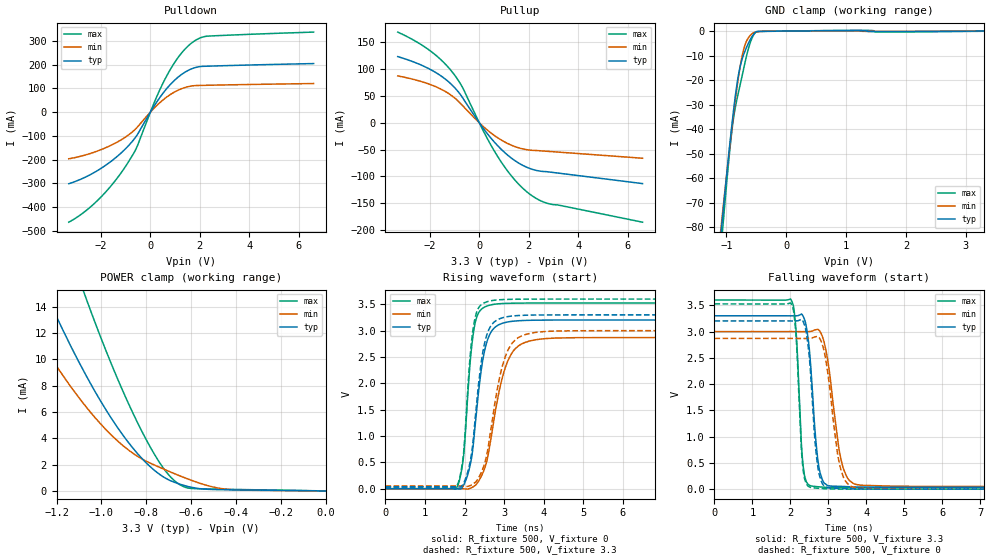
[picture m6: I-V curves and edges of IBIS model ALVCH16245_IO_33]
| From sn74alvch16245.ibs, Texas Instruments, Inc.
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[Model]   ALVCH16245_IO_33
Model_type  I/O
Vinl=0.8
Vinh=2.0
Enable   Active-Low
Vref =   0
Rref =   500
Cref =   50p
Vmeas =   1.5
| variable   typ   min   max
C_comp   8.05pF   6.87pF   9.23pF
| C_pullup   9.24pF   7.49pF   10.37pF
| C_pulldown   11.78pF   9.38pF   15.22pF
| C_tri-state   8.05pF   6.87pF   9.23pF
[Temperature Range]   40   100   -40
| Ambient temperature   25   85   -40
[Voltage range]   3.3   3   3.6
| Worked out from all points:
|   slope of the pulldown table from 0 to 0.495 V, typ, clamps not added: 6.36 ohm
|   slope of the pullup table from 0 to 0.495 V, typ, clamps not added: 16.5 ohm
|   GND clamp passes 1 mA (typ) near -0.54 V on its own axis
|   POWER clamp passes 1 mA (typ) near -0.72 V on its own axis
|   rising waveform, R_fixture 500, V_fixture 0: 20-80 % time 302ps typ, 451ps min, 214ps max; typ from 0 V to 3.2 V
|   falling waveform, R_fixture 500, V_fixture 3.3: 20-80 % time 202ps typ, 319ps min, 140ps max; typ from 3.3 V to 0.037 V
|   rising waveform, R_fixture 500, V_fixture 3.3: 20-80 % time 293ps typ, 428ps min, 207ps max; typ from 0.037 V to 3.3 V
|   falling waveform, R_fixture 500, V_fixture 0: 20-80 % time 193ps typ, 300ps min, 137ps max; typ from 3.2 V to 0 V
[GND Clamp]
| ALVCH16245_IO_33
|   Voltage   I(typ)   I(min)   I(max)
-3.3V     -724.5mA   -661.5mA   -819.8mA
-1.105V   -86.29mA   -83.67mA   -93.18mA
-1.08V    -79.83mA   -77.81mA   -85.86mA
-1.06V    -74.72mA   -73.17mA   -80.07mA
-915mV    -39.73mA   -41.03mA   -42.12mA
-865mV    -29.19mA   -30.91mA   -33.08mA
-805mV    -18.81mA   -19.95mA   -25.69mA
-750mV    -12.49mA   -11.73mA   -19.65mA
-690mV    -8.181mA   -5.715mA   -12.93mA
-545mV    -1.258mA   -688uA     -1.566mA
-315mV    -79.54uA   -56.38uA   -115.7uA
3.3V      119.8pA    41.63uA    -79.23uA
[POWER Clamp]
| ALVCH16245_IO_33
|   Voltage   I(typ)   I(min)   I(max)
-3.3V     128.4mA    96.51mA    173.7mA
-1.385V   20.52mA    14.71mA    31.41mA
-1.235V   14.54mA    10.41mA    23.02mA
-1.1V     9.791mA    7.084mA    16.15mA
-1.065V   8.672mA    6.321mA    14.48mA
-960mV    5.636mA    4.319mA    9.831mA
-860mV    3.263mA    2.869mA    5.931mA
-750mV    1.378mA    1.864mA    2.4mA
-665mV    600.8uA    1.246mA    642.9uA
-600mV    278.6uA    814uA      185.8uA
-450mV    90.53uA    139.8uA    126uA
-48.03fV  119.8pA    370.9pA    68.2pA
[Pulldown]
| ALVCH16245_IO_33
|   Voltage   I(typ)   I(min)   I(max)
-3.3V     -301.6mA   -196.5mA   -463.9mA
-2.73V    -278.9mA   -183.5mA   -425.6mA
-2.155V   -247.3mA   -164.4mA   -374.1mA
-1.6V     -208.1mA   -140mA     -311.9mA
-1.085V   -162.5mA   -110.4mA   -241.1mA
-570mV    -101.4mA   -67.91mA   -152.4mA
185mV     31.43mA    20.51mA    47.78mA
670mV     100.6mA    64.5mA     154.8mA
1.17V     151.9mA    95.01mA    237.4mA
1.67V     182.8mA    110.5mA    291.9mA
2.31V     194mA      113.5mA    320.7mA
6.6V      205mA      120.8mA    337.8mA
[Pullup]
| ALVCH16245_IO_33
|   Voltage   I(typ)   I(min)   I(max)
-3.3V     123.5mA    87.44mA    169.1mA
-2.045V   101mA      72.4mA     136.2mA
-1.55V    87.39mA    62.74mA    117.4mA
-1.13V    71.66mA    51.07mA    96.68mA
-685mV    47.27mA    32.42mA    66.38mA
180mV     -11.59mA   -7.766mA   -16.76mA
760mV     -43.54mA   -28.44mA   -64.12mA
1.38V     -68.63mA   -43.29mA   -103.6mA
2V        -84.39mA   -50.65mA   -131.6mA
2.405V    -89.66mA   -51.96mA   -143.6mA
2.81V     -91.58mA   -53.32mA   -150.8mA
6.6V      -113.3mA   -66.05mA   -185.3mA
[Ramp]
| ALVCH16245_IO_33
| variable   typ   min   max
dV/dt_r   1.93/3.05E-10   1.73/4.66E-10   2.12/2.19E-10
dV/dt_f   1.98/2.07E-10   1.79/3.36E-10   2.16/1.47E-10
R_load = 500
[Rising Waveform]
| ALVCH16245_IO_33
R_fixture =   500
C_fixture =   0
L_fixture =   0
V_fixture =   0
V_fixture_min = 0
V_fixture_max = 0
|   Time   V(typ)   V(min)   V(max)
0s        395.9pV    1.295nV    284.2pV
1.8ns     -1.185mV   2.216mV    18.92mV
1.965ns   51.97mV    -984uV     549.4mV
2.145ns   463.4mV    9.047mV    2.435V
2.27ns    1.222V     63.64mV    3.156V
2.515ns   2.649V     403.8mV    3.451V
2.835ns   3.1V       1.702V     3.509V
3.275ns   3.183V     2.652V     3.522V
4.31ns    3.202V     2.86V      3.526V
50ns      3.202V     2.869V     3.526V
[Falling Waveform]
| ALVCH16245_IO_33
R_fixture =   500
C_fixture =   0
L_fixture =   0
V_fixture =   3.3
V_fixture_min = 3
V_fixture_max = 3.6
|   Time   V(typ)   V(min)   V(max)
0s        3.3V       3V         3.6V
2.025ns   3.299V     3V         3.599V
2.15ns    3.3V       2.999V     3.032V
2.355ns   3.266V     2.998V     348mV
2.5ns     2.678V     2.999V     77.32mV
2.69ns    799.5mV    3.037V     48.91mV
2.95ns    86.06mV    2.603V     35.22mV
3.38ns    51.7mV     439.6mV    28.37mV
3.86ns    40.4mV     74.47mV    27.08mV
50ns      37.01mV    51.2mV     26.69mV
[Rising Waveform]
| ALVCH16245_IO_33
R_fixture =   500
C_fixture =   0
L_fixture =   0
V_fixture =   3.3
V_fixture_min = 3
V_fixture_max = 3.6
|   Time   V(typ)   V(min)   V(max)
0s        37.01mV    51.2mV     26.69mV
1.8ns     35.43mV    52.78mV    46.2mV
1.965ns   91.67mV    49.31mV    597.5mV
2.135ns   492.5mV    58.04mV    2.465V
2.25ns    1.181V     109mV      3.187V
2.49ns    2.707V     440.8mV    3.526V
2.815ns   3.2V       1.838V     3.583V
3.235ns   3.281V     2.791V     3.596V
4.235ns   3.299V     2.992V     3.6V
50ns      3.3V       3V         3.6V
[Falling Waveform]
| ALVCH16245_IO_33
R_fixture =   500
C_fixture =   0
L_fixture =   0
V_fixture =   0
V_fixture_min = 0
V_fixture_max = 0
|   Time   V(typ)   V(min)   V(max)
0s        3.202V     2.869V     3.526V
2.02ns    3.201V     2.869V     3.531V
2.15ns    3.203V     2.868V     2.934V
2.335ns   3.194V     2.868V     394mV
2.5ns     2.526V     2.869V     44.1mV
2.64ns    1.015V     2.897V     23.06mV
2.91ns    57.49mV    2.559V     8.667mV
3.33ns    13.85mV    380.8mV    1.617mV
3.755ns   3.616mV    22.6mV     447.1uV
50ns      186.2nV    331.3nV    91.75nV
